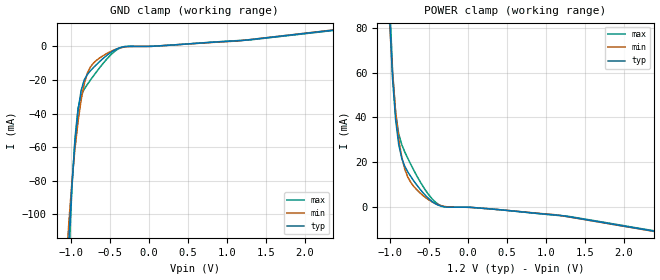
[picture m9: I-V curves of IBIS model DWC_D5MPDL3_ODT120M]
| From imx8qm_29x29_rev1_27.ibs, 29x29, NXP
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[Model] DWC_D5MPDL3_ODT120M
Model_type   Input
Polarity   Non-Inverting
Enable   Active-High
C_comp   1.461pF   1.367pF   1.572pF
C_comp_power_clamp   339.867fF   312.518fF   361.854fF
C_comp_gnd_clamp 1.088pF   1.012pF   1.186pF
Vinh = 735.000mV
Vinl = 465.000mV
[Model Spec]
D_overshoot_ampl_h 0.35 NA   NA
D_overshoot_ampl_l 0.35 NA   NA
D_overshoot_area_l 100.000p NA   NA
D_overshoot_area_h 100.000p NA   NA
[Receiver Thresholds]
Vcross_low = 480.000mV
Vcross_high = 720.000mV
Vdiff_ac = 270.000mV
Vdiff_dc = 200.000mV
Tdiffslew_ac = 10.000ns
[Temperature Range]   25.000   125.000   -40.000
[Voltage Range]   1.200V   1.140V   1.300V
[GND Clamp Reference]   0.00V   0.00V   0.00V
[C Comp Corner]
| variable   typ   min   max
C_comp 1.461pF   1.572pF   1.367pF
C_comp_pullup 339.867fF   361.854fF   312.518fF
C_comp_pulldown 1.088pF   1.186pF   1.012pF
[POWER Clamp Reference]   1.200V   1.140V   1.300V
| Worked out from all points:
|   GND clamp passes 1 mA (typ) near -0.38 V on its own axis
|   POWER clamp passes 1 mA (typ) near -0.39 V on its own axis
[GND Clamp]
-1.182V   -340.1mA   -253.2mA   -429.8mA
-1.064V   -158.7mA   -134.2mA   -183.2mA
-1.024V   -116.1mA   -105mA     -126.7mA
-984.8mV  -82.66mA   -80.81mA   -84.56mA
-945.5mV  -57.01mA   -60.94mA   -54.8mA
-906.1mV  -38.22mA   -44.74mA   -36.93mA
-866.7mV  -26.21mA   -31.87mA   -29.1mA
-787.9mV  -16.73mA   -16.05mA   -22.68mA
-630.3mV  -9.021mA   -6.886mA   -12.71mA
-433.3mV  -2.02mA    -1.859mA   -2.786mA
-315.2mV  -118.5uA   -336.7uA   -76.04uA
2.364V    9.738mA    9.839mA    9.516mA
[Power Clamp]
-1.164V   308.3mA    238.8mA    377.2mA
-1.006V   86.46mA    83.39mA    94.14mA
-966.7mV  57.41mA    59.53mA    60.9mA
-927.3mV  39.01mA    42.29mA    42.22mA
-887.9mV  28.02mA    30.34mA    32.76mA
-848.5mV  21.79mA    22.23mA    27.87mA
-809.1mV  18.16mA    16.85mA    24.57mA
-730.3mV  13.5mA     10.89mA    18.89mA
-533.3mV  4.814mA    4.011mA    6.991mA
-297mV    98.84uA    285.2uA    145.7uA
1.2V      -3.735mA   -3.816mA   -3.837mA
2.382V    -10.73mA   -10.81mA   -10.52mA
